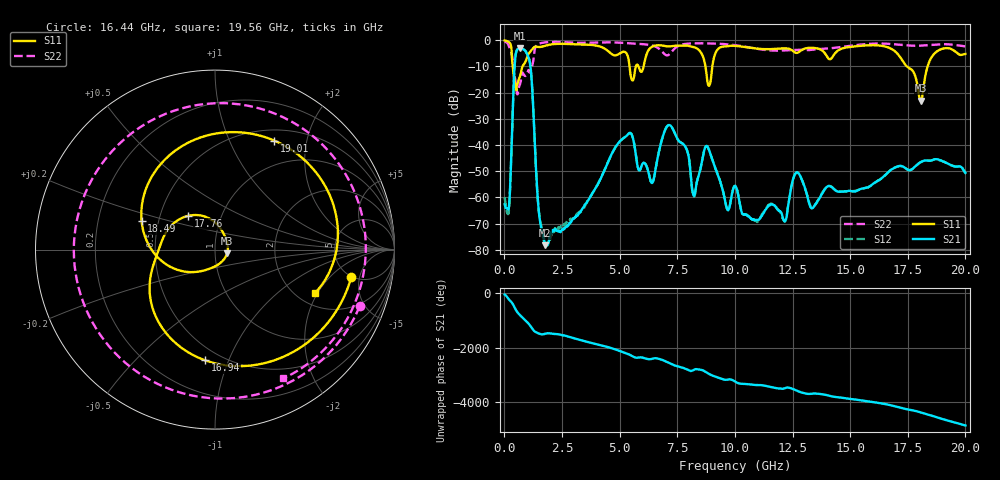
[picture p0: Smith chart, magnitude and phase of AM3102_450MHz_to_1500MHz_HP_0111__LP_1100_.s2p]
!Agilent Technologies,E8364B,MY43040894,A.07.50.67
!Agilent E8364B: A.07.50.67
!Date: Thursday, January 11, 2018 05:54:16
!Correction: S11(Full 2 Port(1,2))
!S21(Full 2 Port(1,2))
!S12(Full 2 Port(1,2))
!S22(Full 2 Port(1,2))
!S2P File: Measurements: S11, S21, S12, S22:
# Hz S  dB  R 50
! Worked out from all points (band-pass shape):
!   1601 points, 10 MHz to 20 GHz, reference 50 ohm
!   highest |S21| = -3.10 dB at 672.2 MHz (marker M1); lowest = -78.4 dB at 1.772 GHz (marker M2)
!   |S21| within 3 dB of the highest: 481.2 MHz to 1.03 GHz (548.9 MHz wide, 72.6 % of centre)
!   lowest |S11| = -23.0 dB at 18.06 GHz (marker M3), VSWR 1.15, Z = 57.2 - j2.41 ohm
!   |S11| at or under -10 dB: 362.5 MHz to 785.4 MHz (422.8 MHz wide, 73.7 % of centre); 8.723 GHz to 9.021 GHz (297.7 MHz wide, 3.36 % of centre); 17.47 GHz to 18.36 GHz (892.7 MHz wide, 4.98 % of centre)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
!   |S22| runs from -20.7 to -0.5 dB; largest |S21 - S12| = 0.0019
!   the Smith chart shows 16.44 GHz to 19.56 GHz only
!   S11 on the Smith chart (normalised r, x): 16.44 GHz: 4.90, -3.77; 16.94 GHz: 0.41, -0.83; 17.76 GHz: 0.70, +0.28; 18.49 GHz: 0.40, +0.16; 19.01 GHz: 0.64, +1.48; 19.56 GHz: 2.50, -1.90
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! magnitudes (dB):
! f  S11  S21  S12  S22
! 10 MHz  -0.1  -62.6  -60.0  -0.5
! 184.9 MHz  -0.7  -64.7  -66.0  -1.9
! 459.8 MHz  -16.7  -8.0  -8.0  -14.5
! 672.2 MHz  -13.9  -3.1  -3.1  -16.9
! 1.109 GHz  -4.5  -8.7  -8.7  -12.3
! 1.484 GHz  -2.6  -64.4  -64.4  -1.4
! 1.772 GHz  -2.1  -78.4  -77.6  -0.8
! 3.346 GHz  -1.6  -64.8  -65.2  -1.0
! 5.37 GHz  -6.6  -35.8  -35.8  -1.1
! 6.682 GHz  -1.9  -43.4  -43.5  -3.0
! 8.881 GHz  -17.4  -41.9  -41.9  -1.2
! 10.01 GHz  -2.1  -55.6  -55.6  -1.9
! 13.34 GHz  -2.9  -64.2  -64.0  -3.6
! 16.44 GHz  -2.2  -52.1  -52.1  -1.3
! 16.68 GHz  -2.8  -50.2  -50.2  -1.4
! 16.94 GHz  -4.2  -48.7  -48.6  -1.5
! 17.76 GHz  -12.4  -48.7  -48.6  -2.1
! 18.06 GHz  -23.0  -46.5  -46.5  -2.0
! 18.49 GHz  -7.2  -46.0  -46.0  -1.8
! 19.01 GHz  -3.2  -46.2  -46.1  -1.5
! 19.56 GHz  -4.3  -48.2  -48.1  -1.8
! 20 GHz  -5.2  -50.6  -50.8  -2.3
